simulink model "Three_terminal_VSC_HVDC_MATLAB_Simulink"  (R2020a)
settings: Solver=ode4  StartTime=0.0  StopTime=Tstop  MaxStep=1e-4  RelTol=1e-3
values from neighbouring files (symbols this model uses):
  kw = 5    [Parameterisation_Three_terminal_VSC_HVDC_MATLAB_Simulink.m]
undefined symbols (not defined in the file or in its folder): bridge, phase, pulses, Sim, Three, VSC1, VSC123, VSC2, VSC3
libraries: powerlib x70, powerlib_meascontrol x9, simulink x3
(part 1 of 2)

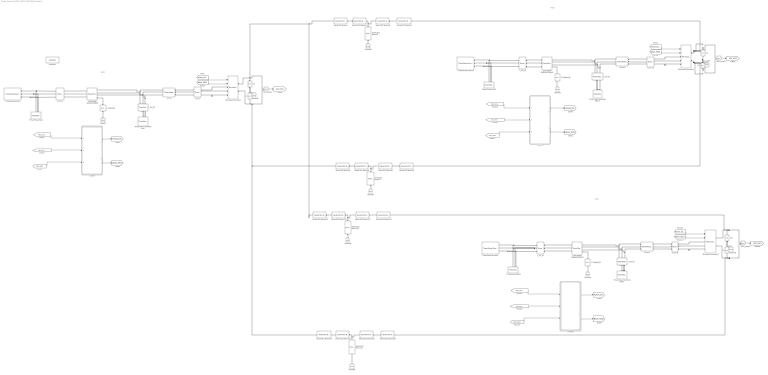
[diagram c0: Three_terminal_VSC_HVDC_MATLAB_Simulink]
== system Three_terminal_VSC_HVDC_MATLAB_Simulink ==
  note: VSC2
  note: VSC3
  note: VSC1
  1.0 [Mohm] : powerlib/Elements/Series RLC Branch  LConnTagsString=__new0  RConnTagsString=__new0  BranchType=R  Resistance=1e6  Inductance=1e-3  SetiL0=off  InitialCurrent=0  Capacitance=1e-6  Setx0=off  InitialVoltage=0  Measurements=None
  1.0 [Mohm]1 : powerlib/Elements/Series RLC Branch  LConnTagsString=__new0  RConnTagsString=__new0  BranchType=R  Resistance=1e6  Inductance=1e-3  SetiL0=off  InitialCurrent=0  Capacitance=1e-6  Setx0=off  InitialVoltage=0  Measurements=None
  1.0 [Mohm]2 : powerlib/Elements/Series RLC Branch  LConnTagsString=__new0  RConnTagsString=__new0  BranchType=R  Resistance=1e6  Inductance=1e-3  SetiL0=off  InitialCurrent=0  Capacitance=1e-6  Setx0=off  InitialVoltage=0  Measurements=None
  1500 [MVA] 420[kV]/230[kV : powerlib/Elements/Three-Phase Transformer (Two Windings)  Winding1Connection=Yg  Winding2Connection=Yn  CoreType=Five-limb core (shell-type)  SetSaturation=off  Hysteresis=off  DataFile='hysteresis'  SetInitialFlux=off  Measurements=None  UNITS=pu  NominalPower=[VSC1.Trf.nominal.MVA,VSC1.Trf.nominal.f]  Winding1=[VSC1.Trf.nominal.HV VSC1.Trf.ur VSC1.Trf.uk]  Winding2=[VSC1.Trf.nominal.LV VSC1.Trf.ur VSC1.Trf.uk]  Rm=VSC1.Trf.MagRm  Lm=VSC1.Trf.MagXm  L0=1.6029  Saturation=[0 0;0.0024 1.2;1 1.52]  InitialFluxes=[0.00087946 -0.00087946 0.00076952]  BreakLoop=off  DiscreteSolver=Trapezoidal iterative  DataType=off  TransfoNumber=1
  1500 [MVA] 420[kV]/230[kV1 : powerlib/Elements/Three-Phase Transformer (Two Windings)  Winding1Connection=Yg  Winding2Connection=Yn  CoreType=Five-limb core (shell-type)  SetSaturation=off  Hysteresis=off  DataFile='hysteresis'  SetInitialFlux=off  Measurements=None  UNITS=pu  NominalPower=[VSC1.Trf.nominal.MVA,VSC2.Trf.nominal.f]  Winding1=[VSC1.Trf.nominal.HV VSC1.Trf.ur VSC1.Trf.uk]  Winding2=[VSC1.Trf.nominal.LV VSC1.Trf.ur VSC1.Trf.uk]  Rm=VSC1.Trf.MagRm  Lm=VSC1.Trf.MagXm  L0=1.6029  Saturation=[0 0;0.0024 1.2;1 1.52]  InitialFluxes=[0.00087946 -0.00087946 0.00076952]  BreakLoop=off  DiscreteSolver=Trapezoidal iterative  DataType=off  TransfoNumber=1
  1500 [MVA] 420[kV]/230[kV2 : powerlib/Elements/Three-Phase Transformer (Two Windings)  Winding1Connection=Yg  Winding2Connection=Yn  CoreType=Five-limb core (shell-type)  SetSaturation=off  Hysteresis=off  DataFile='hysteresis'  SetInitialFlux=off  Measurements=None  UNITS=pu  NominalPower=[VSC1.Trf.nominal.MVA,VSC2.Trf.nominal.f]  Winding1=[VSC3.Trf.nominal.HV VSC1.Trf.ur VSC1.Trf.uk]  Winding2=[VSC1.Trf.nominal.LV VSC1.Trf.ur VSC1.Trf.uk]  Rm=VSC1.Trf.MagRm  Lm=VSC1.Trf.MagXm  L0=1.6029  Saturation=[0 0;0.0024 1.2;1 1.52]  InitialFluxes=[0.00087946 -0.00087946 0.00076952]  BreakLoop=off  DiscreteSolver=Trapezoidal iterative  DataType=off  TransfoNumber=1
  C/1 : powerlib/Elements/Series RLC Branch  LConnTagsString=__new0  RConnTagsString=__new0  BranchType=C  Resistance=0.000001  Inductance=1e-3  SetiL0=off  InitialCurrent=0  Capacitance=VSC1.Capacitor  Setx0=on  InitialVoltage=200e3  Measurements=None
  C/2 : powerlib/Elements/Series RLC Branch  LConnTagsString=__new0  RConnTagsString=__new0  BranchType=RC  Resistance=1e-12  Inductance=1e-3  SetiL0=off  InitialCurrent=0  Capacitance=VSC1.Capacitor  Setx0=on  InitialVoltage=200e3  Measurements=None
  C/3 : powerlib/Elements/Series RLC Branch  LConnTagsString=__new0  RConnTagsString=__new0  BranchType=C  Resistance=0.000001  Inductance=1e-3  SetiL0=off  InitialCurrent=0  Capacitance=VSC1.Capacitor  Setx0=on  InitialVoltage=200e3  Measurements=None
  C/4 : powerlib/Elements/Series RLC Branch  LConnTagsString=__new0  RConnTagsString=__new0  BranchType=RC  Resistance=1e-12  Inductance=1e-3  SetiL0=off  InitialCurrent=0  Capacitance=VSC1.Capacitor  Setx0=on  InitialVoltage=200e3  Measurements=None
  C/5 : powerlib/Elements/Series RLC Branch  LConnTagsString=__new0  RConnTagsString=__new0  BranchType=C  Resistance=0.000001  Inductance=1e-3  SetiL0=off  InitialCurrent=0  Capacitance=VSC1.Capacitor  Setx0=on  InitialVoltage=200e3  Measurements=None
  C/6 : powerlib/Elements/Series RLC Branch  LConnTagsString=__new0  RConnTagsString=__new0  BranchType=RC  Resistance=1e-12  Inductance=1e-3  SetiL0=off  InitialCurrent=0  Capacitance=VSC1.Capacitor  Setx0=on  InitialVoltage=200e3  Measurements=None
  Control : Subsystem
  Control1 : Subsystem
  Control2 : Subsystem
  Ground{,1..9} (10 alike) : powerlib/Elements/Ground  LConnTagsString=a
  I_C/V_C : powerlib/Measurements/Three-Phase V-I Measurement  VoltageMeasurement=no  SetLabelV=off  LabelV=Vabc_converter  Vpu=off  VpuLL=off  CurrentMeasurement=yes  SetLabelI=on  LabelI=Iabc_converter_VSC1  Ipu=off  Pbase=100e6  Vbase=500e3  OutputType=Complex  PhasorSimulation=off  PSBequivalent=0
  I_C/V_C1 : powerlib/Measurements/Three-Phase V-I Measurement  VoltageMeasurement=phase-to-ground  SetLabelV=on  LabelV=Vabc_filter  Vpu=off  VpuLL=off  CurrentMeasurement=yes  SetLabelI=on  LabelI=Iabc_filter  Ipu=off  Pbase=100e6  Vbase=500e3  OutputType=Complex  PhasorSimulation=off  PSBequivalent=0
  I_C/V_C2 : powerlib/Measurements/Three-Phase V-I Measurement  VoltageMeasurement=no  SetLabelV=off  LabelV=Vabc_converter  Vpu=off  VpuLL=off  CurrentMeasurement=yes  SetLabelI=on  LabelI=Iabc_converter_VSC2  Ipu=off  Pbase=100e6  Vbase=500e3  OutputType=Complex  PhasorSimulation=off  PSBequivalent=0
  I_C/V_C3 : powerlib/Measurements/Three-Phase V-I Measurement  VoltageMeasurement=no  SetLabelV=off  LabelV=Vabc_filter  Vpu=off  VpuLL=off  CurrentMeasurement=no  SetLabelI=off  LabelI=Iabc_filter  Ipu=off  Pbase=100e6  Vbase=500e3  OutputType=Complex  PhasorSimulation=off  PSBequivalent=0
  I_C/V_C4 : powerlib/Measurements/Three-Phase V-I Measurement  VoltageMeasurement=no  SetLabelV=off  LabelV=Vabc_converter  Vpu=off  VpuLL=off  CurrentMeasurement=yes  SetLabelI=on  LabelI=Iabc_converter_VSC3  Ipu=off  Pbase=100e6  Vbase=500e3  OutputType=Complex  PhasorSimulation=off  PSBequivalent=0
  I_C/V_C5 : powerlib/Measurements/Three-Phase V-I Measurement  VoltageMeasurement=no  SetLabelV=off  LabelV=Vabc_filter  Vpu=off  VpuLL=off  CurrentMeasurement=no  SetLabelI=off  LabelI=Iabc_filter  Ipu=off  Pbase=100e6  Vbase=500e3  OutputType=Complex  PhasorSimulation=off  PSBequivalent=0
  I_S/V_S : powerlib/Measurements/Three-Phase V-I Measurement  VoltageMeasurement=phase-to-ground  SetLabelV=on  LabelV=Vabc_source_VSC1  Vpu=off  VpuLL=off  CurrentMeasurement=yes  SetLabelI=on  LabelI=Iabc_source_VSC1  Ipu=off  Pbase=100e6  Vbase=500e3  OutputType=Complex  PhasorSimulation=off  PSBequivalent=0
  I_S/V_S1 : powerlib/Measurements/Three-Phase V-I Measurement  VoltageMeasurement=phase-to-ground  SetLabelV=on  LabelV=Vabc_source_VSC2  Vpu=off  VpuLL=off  CurrentMeasurement=yes  SetLabelI=on  LabelI=Iabc_source_VSC2  Ipu=off  Pbase=100e6  Vbase=500e3  OutputType=Complex  PhasorSimulation=off  PSBequivalent=0
  I_S/V_S2 : powerlib/Measurements/Three-Phase V-I Measurement  VoltageMeasurement=phase-to-ground  SetLabelV=on  LabelV=Vabc_source_VSC3  Vpu=off  VpuLL=off  CurrentMeasurement=yes  SetLabelI=on  LabelI=Iabc_source_VSC3  Ipu=off  Pbase=100e6  Vbase=500e3  OutputType=Complex  PhasorSimulation=off  PSBequivalent=0
  LfConv : powerlib/Elements/Three-Phase Series RLC Branch  LConnTagsString=A|B|C  RConnTagsString=A|B|C  BranchType=L  Resistance=1  Inductance=VSC1.SeriesFilter.Lf  Capacitance=1e-6  Measurements=None
  LfConv1 : powerlib/Elements/Three-Phase Series RLC Branch  LConnTagsString=A|B|C  RConnTagsString=A|B|C  BranchType=L  Resistance=1  Inductance=VSC1.SeriesFilter.Lf  Capacitance=1e-6  Measurements=None
  LfConv2 : powerlib/Elements/Three-Phase Series RLC Branch  LConnTagsString=A|B|C  RConnTagsString=A|B|C  BranchType=L  Resistance=1  Inductance=VSC1.SeriesFilter.Lf  Capacitance=1e-6  Measurements=None
  Series RLC Branch{,3,5,8,10,13,15,18} (8 alike) : powerlib/Elements/Series RLC Branch  LConnTagsString=__new0  RConnTagsString=__new0  BranchType=R  Resistance=VSC123.Rline  Inductance=1e-3  SetiL0=off  InitialCurrent=0  Capacitance=1e-6  Setx0=off  InitialVoltage=0  Measurements=None
  Series RLC Branch{1,4,6,9,11,14,16,19} (8 alike) : powerlib/Elements/Series RLC Branch  LConnTagsString=__new0  RConnTagsString=__new0  BranchType=L  Resistance=VSC123.Rline  Inductance=VSC123.Lline  SetiL0=off  InitialCurrent=0  Capacitance=1e-6  Setx0=off  InitialVoltage=0  Measurements=None
  Series RLC Branch{2,7,12,17} (4 alike) : powerlib/Elements/Series RLC Branch  LConnTagsString=__new0  RConnTagsString=__new0  BranchType=C  Resistance=VSC123.Rline  Inductance=VSC123.Lline  SetiL0=off  InitialCurrent=0  Capacitance=VSC123.Cline  Setx0=off  InitialVoltage=0  Measurements=None
  Three-Phase Harmonic Filter : powerlib/Elements/Three-Phase Harmonic Filter  LConnTagsString=A|B|C  FilterType=High-pass  FilterConnection=Y (grounded)  ParNom=[230e3 60]  Qc=75e6  Fr=[450]  Frd=[11*60 13*60]  Q=0.08  Measurements=None
  Three-Phase Harmonic Filter1 : powerlib/Elements/Three-Phase Harmonic Filter  LConnTagsString=A|B|C  FilterType=High-pass  FilterConnection=Y (grounded)  ParNom=[230e3 50]  Qc=75e6  Fr=[450]  Frd=[11*60 13*60]  Q=0.08  Measurements=None
  Three-Phase Harmonic Filter2 : powerlib/Elements/Three-Phase Harmonic Filter  LConnTagsString=A|B|C  FilterType=High-pass  FilterConnection=Y (grounded)  ParNom=[230e3 50]  Qc=75e6  Fr=[450]  Frd=[11*60 13*60]  Q=0.08  Measurements=None
  Three-Phase Fault : powerlib/Elements/Three-Phase Fault  InitialStates=0  FaultA=on  FaultB=on  FaultC=off  GroundFault=on  SwitchTimes="[VSC1.flt.On  VSC1.flt.Off]"  External=off  SwitchStatus=NaN  FaultResistance=VSC1.flt.OnR  GroundResistance=VSC1.flt.GroundR  SnubberResistance=1e6  SnubberCapacitance=inf  Measurements=Fault voltages and currents
  Three-Phase Fault1 : powerlib/Elements/Three-Phase Fault  InitialStates=0  FaultA=on  FaultB=on  FaultC=on  GroundFault=on  SwitchTimes="[VSC2.flt.On  VSC2.flt.Off]"  External=off  SwitchStatus=NaN  FaultResistance=VSC1.flt.OnR  GroundResistance=VSC1.flt.GroundR  SnubberResistance=1e6  SnubberCapacitance=inf  Measurements=Fault voltages and currents
  Three-Phase Fault2 : powerlib/Elements/Three-Phase Fault  InitialStates=0  FaultA=on  FaultB=on  FaultC=on  GroundFault=on  SwitchTimes="[VSC3.flt.On  VSC3.flt.Off]"  External=off  SwitchStatus=NaN  FaultResistance=VSC1.flt.OnR  GroundResistance=VSC1.flt.GroundR  SnubberResistance=1e6  SnubberCapacitance=inf  Measurements=Fault voltages and currents
  Three-Phase Source : powerlib/Electrical Sources/Three-Phase Source  InternalConnection=Yg  VoltagePhases=off  Voltage=VSC1.source.nominal.v  PhaseAngle=VSC1.source.nominal.theta  Voltage_phases=[25e3 25e3 25e3]/sqrt(3)  PhaseAngles_phases=[0 -120 +120]  Frequency=VSC1.source.nominal.f  NonIdealSource=on  SpecifyImpedance=off  Resistance=VSC1.source.nominal.r  Inductance=VSC1.source.nominal.l  ShortCircuitLevel=100e6  BaseVoltage=VSC1.source.basevoltage  XRratio=7  BusType=swing  Pref=10e3  Qref=0  Prefabc=[10e3, 10e3, 10e3]  Qrefabc=[0, 0, 0]  Qmin=-inf  Qmax=inf
  Three-Phase Source1 : powerlib/Electrical Sources/Three-Phase Source  InternalConnection=Yg  VoltagePhases=off  Voltage=VSC1.source.nominal.v  PhaseAngle=VSC1.source.nominal.theta  Voltage_phases=[25e3 25e3 25e3]/sqrt(3)  PhaseAngles_phases=[0 -120 +120]  Frequency=VSC2.source.nominal.f  NonIdealSource=on  SpecifyImpedance=off  Resistance=VSC1.source.nominal.r  Inductance=VSC2.source.nominal.l  ShortCircuitLevel=100e6  BaseVoltage=VSC1.source.basevoltage  XRratio=7  BusType=swing  Pref=10e3  Qref=0  Prefabc=[10e3, 10e3, 10e3]  Qrefabc=[0, 0, 0]  Qmin=-inf  Qmax=inf
  Three-Phase Source2 : powerlib/Electrical Sources/Three-Phase Source  InternalConnection=Yg  VoltagePhases=off  Voltage=VSC3.source.nominal.v  PhaseAngle=VSC1.source.nominal.theta  Voltage_phases=[25e3 25e3 25e3]/sqrt(3)  PhaseAngles_phases=[0 -120 +120]  Frequency=VSC2.source.nominal.f  NonIdealSource=on  SpecifyImpedance=off  Resistance=VSC1.source.nominal.r  Inductance=VSC2.source.nominal.l  ShortCircuitLevel=100e6  BaseVoltage=VSC3.source.nominal.v  XRratio=7  BusType=swing  Pref=10e3  Qref=0  Prefabc=[10e3, 10e3, 10e3]  Qrefabc=[0, 0, 0]  Qmin=-inf  Qmax=inf
  Two-Level Converter : powerlib/Power Electronics/Two-Level Converter  ModelType=Switching devices  Ron=0.005  Rs=1e6  Cs=inf  Vforward=[0,0]  Ron_Diode=1e-3  Rs_Diode=1e6  Cs_Diode=inf  Vf_Diode=1e-3  Rs_CurrentSource=inf
  Two-Level Converter1 : powerlib/Power Electronics/Two-Level Converter  ModelType=Switching devices  Ron=0.005  Rs=1e6  Cs=inf  Vforward=[0,0]  Ron_Diode=1e-3  Rs_Diode=1e6  Cs_Diode=inf  Vf_Diode=1e-3  Rs_CurrentSource=inf
  Two-Level Converter2 : powerlib/Power Electronics/Two-Level Converter  ModelType=Switching devices  Ron=0.005  Rs=1e6  Cs=inf  Vforward=[0,0]  Ron_Diode=1e-3  Rs_Diode=1e6  Cs_Diode=inf  Vf_Diode=1e-3  Rs_CurrentSource=inf
  UDC_meas : powerlib/Measurements/Voltage Measurement  PhasorSimulation=off  OutputType=Complex  PSBequivalent=0
  UDC_meas1 : powerlib/Measurements/Voltage Measurement  PhasorSimulation=off  OutputType=Complex  PSBequivalent=0
  UDC_meas2 : powerlib/Measurements/Voltage Measurement  PhasorSimulation=off  OutputType=Complex  PSBequivalent=0
  powergui : powerlib/powergui  Priority=1  SimulationMode=Discrete  SampleTime=Sim.Ts  frequency=60  Iterations=50  frequencyindice=0  Pbase=100e6  ErrMax=1e-4  UnitsV=kV  UnitsW=MW  buscounter=0  FunctionMessages=off  echomessages=off  EnableUseOfTLC=off  CurrentSourceSwitches=off  DisableSnubberDevices=off  DisableRonSwitches=off  DisableVfSwitches=off  DisplayEquations=off  AutomaticDiscreteSolvers=off  SolverType=Tustin/Backward Euler (TBE)  Interpol=off  ExternalGateDelay=off  methode=off  Ts=100  x0status=blocks  SPID=on  SwTol=0  HookPort=off  NonlinearTolerance=1e-4  nMaxIteration=100  ContinueOnMaxIteration=off  RestoreLinks=warning  ResistiveCurrentMeasurement=off  Frange=[0:2:500]  Ylog=off  Xlog=on  ShowGrid=off  save=off  variable=ZData  structure=0  ZoomFFT=off  StartTime=0.0  cycles=1  DisplayStyle=1  fundamental=60  FreqAxis=off  MaxFrequency=1000  frequencyindicesteady=1  RmsSteady=1  display=off
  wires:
  [Vabc_source_VSC1] -> Control/1(Umeas)
  [Iabc_converter_VSC1] -> Control/2(Imeas)
  Control/1(Pulses) -> [Pulses_VSC1]
  [Pulses_VSC1] -> Two-Level Converter/1
  [Block_VSC1] -> Two-Level Converter/2
  UDC_meas/1 -> [UDC_VSC1]
  [UDC_VSC1] -> Control/3(UDC)
  UDC_meas1/1 -> [UDC_VSC2]
  [Vabc_source_VSC2] -> Control1/1(Umeas)
  [Block_VSC2] -> Two-Level Converter1/2
  [UDC_VSC2] -> Control1/3(UDC)
  [Iabc_converter_VSC2] -> Control1/2(Imeas)
  [Pulses_VSC2] -> Two-Level Converter1/1
  Control1/1(Pulses) -> [Pulses_VSC2]
  [Block_VSC3] -> Two-Level Converter2/2
  UDC_meas2/1 -> [UDC_VSC3]
  [Vabc_source_VSC3] -> Control2/1(Umeas)
  Control2/2("Block ") -> [Block_VSC3]
  [Pulses_VSC3] -> Two-Level Converter2/1
  Control2/1(Pulses) -> [Pulses_VSC3]
  [Iabc_converter_VSC3] -> Control2/2(Imeas)
  [UDC_VSC3] -> Control2/3(UDC)
  Control1/2("Block ") -> [Block_VSC2]
  Control/2("Block ") -> [Block_VSC1]
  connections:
  1.0 [Mohm]/LConn1 -- 1500 [MVA] 420[kV]/230[kV/RConn4
  Ground/LConn1 -- 1.0 [Mohm]/RConn1
  LfConv/RConn1 -- I_C/V_C/LConn1
  LfConv/RConn2 -- I_C/V_C/LConn2
  LfConv/RConn3 -- I_C/V_C/LConn3
  C/2/LConn1 -- UDC_meas/LConn1 -- Series RLC Branch/LConn1 -- Series RLC Branch10/LConn1 -- Two-Level Converter/RConn1
  I_C/V_C1/RConn2 -- LfConv/LConn2 -- 1500 [MVA] 420[kV]/230[kV/RConn2
  I_C/V_C1/RConn3 -- LfConv/LConn3 -- 1500 [MVA] 420[kV]/230[kV/RConn3
  I_C/V_C1/RConn1 -- LfConv/LConn1 -- 1500 [MVA] 420[kV]/230[kV/RConn1
  C/2/RConn1 -- Ground1/LConn1 -- C/1/LConn1
  Three-Phase Source/RConn1 -- Three-Phase Fault/LConn1 -- I_S/V_S/LConn1
  Three-Phase Source/RConn2 -- Three-Phase Fault/LConn2 -- I_S/V_S/LConn2
  Three-Phase Source/RConn3 -- Three-Phase Fault/LConn3 -- I_S/V_S/LConn3
  Series RLC Branch1/LConn1 -- Series RLC Branch/RConn1
  Series RLC Branch2/LConn1 -- Series RLC Branch3/LConn1 -- Series RLC Branch1/RConn1
  Ground6/LConn1 -- Series RLC Branch2/RConn1
  Series RLC Branch4/LConn1 -- Series RLC Branch3/RConn1
  Series RLC Branch7/LConn1 -- Series RLC Branch8/LConn1 -- Series RLC Branch6/RConn1
  Series RLC Branch9/LConn1 -- Series RLC Branch8/RConn1
  Ground7/LConn1 -- Series RLC Branch7/RConn1
  Series RLC Branch6/LConn1 -- Series RLC Branch5/RConn1
  Series RLC Branch12/LConn1 -- Series RLC Branch13/LConn1 -- Series RLC Branch11/RConn1
  Series RLC Branch14/LConn1 -- Series RLC Branch13/RConn1
  Ground8/LConn1 -- Series RLC Branch12/RConn1
  Series RLC Branch11/LConn1 -- Series RLC Branch10/RConn1
  Series RLC Branch17/LConn1 -- Series RLC Branch18/LConn1 -- Series RLC Branch16/RConn1
  Series RLC Branch19/LConn1 -- Series RLC Branch18/RConn1
  Ground9/LConn1 -- Series RLC Branch17/RConn1
  Series RLC Branch16/LConn1 -- Series RLC Branch15/RConn1
  C/3/LConn1 -- C/4/RConn1 -- Ground3/LConn1
  I_C/V_C3/RConn2 -- LfConv1/LConn2 -- 1500 [MVA] 420[kV]/230[kV1/RConn2
  Two-Level Converter1/RConn2 -- UDC_meas1/LConn2 -- Series RLC Branch9/RConn1 -- C/3/RConn1
  I_C/V_C3/RConn1 -- LfConv1/LConn1 -- 1500 [MVA] 420[kV]/230[kV1/RConn1
  Three-Phase Source1/RConn3 -- Three-Phase Fault1/LConn3 -- I_S/V_S1/LConn3
  Two-Level Converter1/RConn1 -- UDC_meas1/LConn1 -- Series RLC Branch4/RConn1 -- C/4/LConn1
  Three-Phase Source1/RConn2 -- Three-Phase Fault1/LConn2 -- I_S/V_S1/LConn2
  Three-Phase Source1/RConn1 -- Three-Phase Fault1/LConn1 -- I_S/V_S1/LConn1
  I_C/V_C3/RConn3 -- 1500 [MVA] 420[kV]/230[kV1/RConn3 -- LfConv1/LConn3
  LfConv1/RConn2 -- I_C/V_C2/LConn2
  LfConv1/RConn3 -- I_C/V_C2/LConn3
  LfConv1/RConn1 -- I_C/V_C2/LConn1
  Ground2/LConn1 -- 1.0 [Mohm]1/RConn1
  1.0 [Mohm]1/LConn1 -- 1500 [MVA] 420[kV]/230[kV1/RConn4
  C/6/RConn1 -- Ground5/LConn1 -- C/5/LConn1
  UDC_meas2/LConn2 -- Series RLC Branch19/RConn1 -- C/5/RConn1 -- Two-Level Converter2/RConn2
  Three-Phase Source2/RConn1 -- Three-Phase Fault2/LConn1 -- I_S/V_S2/LConn1
  UDC_meas2/LConn1 -- C/6/LConn1 -- Series RLC Branch14/RConn1 -- Two-Level Converter2/RConn1
  I_C/V_C5/RConn1 -- LfConv2/LConn1 -- 1500 [MVA] 420[kV]/230[kV2/RConn1
  Three-Phase Source2/RConn3 -- Three-Phase Fault2/LConn3 -- I_S/V_S2/LConn3
  I_C/V_C5/RConn2 -- LfConv2/LConn2 -- 1500 [MVA] 420[kV]/230[kV2/RConn2
  I_C/V_C5/RConn3 -- LfConv2/LConn3 -- 1500 [MVA] 420[kV]/230[kV2/RConn3
  I_S/V_S2/LConn2 -- Three-Phase Source2/RConn2 -- Three-Phase Fault2/LConn2
  LfConv2/RConn2 -- I_C/V_C4/LConn2
  LfConv2/RConn3 -- I_C/V_C4/LConn3
  1.0 [Mohm]2/LConn1 -- 1500 [MVA] 420[kV]/230[kV2/RConn4
  Ground4/LConn1 -- 1.0 [Mohm]2/RConn1
  LfConv2/RConn1 -- I_C/V_C4/LConn1
  1500 [MVA] 420[kV]/230[kV/LConn1 -- I_S/V_S/RConn1
  1500 [MVA] 420[kV]/230[kV/LConn2 -- I_S/V_S/RConn2
  1500 [MVA] 420[kV]/230[kV/LConn3 -- I_S/V_S/RConn3
  1500 [MVA] 420[kV]/230[kV2/LConn1 -- I_S/V_S2/RConn1
  1500 [MVA] 420[kV]/230[kV2/LConn2 -- I_S/V_S2/RConn2
  1500 [MVA] 420[kV]/230[kV2/LConn3 -- I_S/V_S2/RConn3
  1500 [MVA] 420[kV]/230[kV1/LConn1 -- I_S/V_S1/RConn1
  I_S/V_S1/RConn2 -- 1500 [MVA] 420[kV]/230[kV1/LConn2
  I_S/V_S1/RConn3 -- 1500 [MVA] 420[kV]/230[kV1/LConn3
  Three-Phase Harmonic Filter/LConn1 -- I_C/V_C1/LConn1
  Three-Phase Harmonic Filter/LConn2 -- I_C/V_C1/LConn2
  Three-Phase Harmonic Filter/LConn3 -- I_C/V_C1/LConn3
  Three-Phase Harmonic Filter1/LConn1 -- I_C/V_C3/LConn1
  I_C/V_C3/LConn2 -- Three-Phase Harmonic Filter1/LConn2
  Three-Phase Harmonic Filter1/LConn3 -- I_C/V_C3/LConn3
  Three-Phase Harmonic Filter2/LConn1 -- I_C/V_C5/LConn1
  Three-Phase Harmonic Filter2/LConn2 -- I_C/V_C5/LConn2
  Three-Phase Harmonic Filter2/LConn3 -- I_C/V_C5/LConn3
  UDC_meas/LConn2 -- Series RLC Branch15/LConn1 -- Series RLC Branch5/LConn1 -- C/1/RConn1 -- Two-Level Converter/RConn2
  I_C/V_C/RConn1 -- Two-Level Converter/LConn1
  I_C/V_C/RConn2 -- Two-Level Converter/LConn2
  I_C/V_C/RConn3 -- Two-Level Converter/LConn3
  I_C/V_C2/RConn1 -- Two-Level Converter1/LConn1
  I_C/V_C2/RConn2 -- Two-Level Converter1/LConn2
  I_C/V_C2/RConn3 -- Two-Level Converter1/LConn3
  I_C/V_C4/RConn1 -- Two-Level Converter2/LConn1
  I_C/V_C4/RConn2 -- Two-Level Converter2/LConn2
  I_C/V_C4/RConn3 -- Two-Level Converter2/LConn3

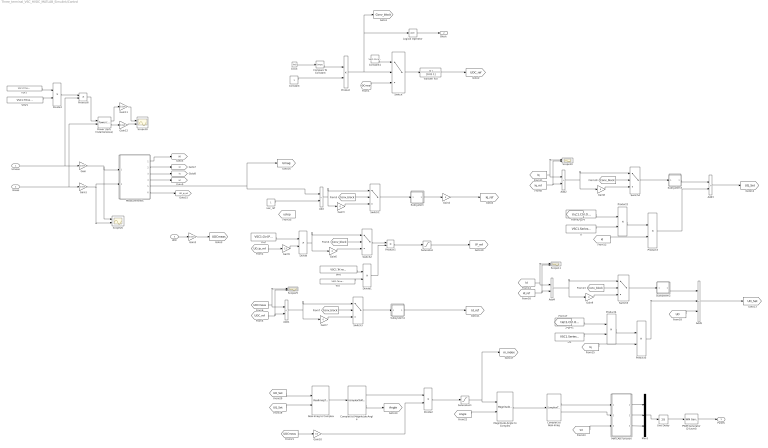
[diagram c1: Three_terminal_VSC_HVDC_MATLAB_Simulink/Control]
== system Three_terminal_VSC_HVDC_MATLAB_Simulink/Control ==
  Umeas : Inport
  Imeas : Inport  Port=2
  UDC : Inport  Port=3
  2*pi*f : Constant  Value=VSC1.Ctrl.Omeganom
  2*pi*f1 : Constant  Value=VSC1.Ctrl.Omeganom
  Add{,1..4} (5 alike) : Sum  Inputs=-+
  Add5 : Sum  Inputs=--+
  Clock : Clock
  Compare To Constant : simulink/Logic and Bit Operations/Compare To Constant  relop=>  const=0.05  OutDataTypeStr=boolean
  Complex to Magnitude-Angle : ComplexToMagnitudeAngle
  Complex to Real-Imag : ComplexToRealImag
  Constant : Constant
  Constant1 : Constant  Value=VSC1.Ctrl.UDCRef_Const
  Divide{,1..3} (4 alike) : Product  Inputs=*/
  Gain : Gain  Gain=1/1e3
  Gain1 : Gain  Gain=1/1e3
  Gain10 : Gain  Gain=0.5
  Gain11 : Gain  Gain=1/1e6
  Gain12 : Gain  Gain=1/1e6
  Gain2 : Gain  Gain=1/1e3
  Gain{3,6..9} (5 alike) : Gain  Gain=0
  Gain4 : Gain
  Gain5 : Gain  Gain=1.5
  Lf : Constant  Value=VSC1.SeriesFilter.Lf
  Lf1 : Constant  Value=VSC1.SeriesFilter.Lf
  Logical Operator : Logic  Operator=NOT  AllPortsSameDT=off  OutDataTypeStr=boolean
  MATLAB Function : MATLAB Function  TreatAsAtomicUnit=on
  Magnitude-Angle to Complex : MagnitudeAngleToComplex
  Measurements : Subsystem
  Mux1 : Mux  Inputs=3
  PWM Generator (2-Level) : powerlib_meascontrol/Pulse & Signal Generators/PWM Generator (2-Level)  ModulatorType=Three-phase bridge (6 pulses)  ModulatorMode=Unsynchronized  Fc=VSC1.Ctrl.fs  Pc=90  nF=33  MinMax="[ -1  1]"  SamplingTechnique=Natural  ModulatingSignals=off  m=0.8  Freq=60  Phase=0  Ts=Sim.Ts  ShowCarrierOutport=off
  "Power (3ph, Instantaneous)" : powerlib_meascontrol/Measurements/Power (3ph, Instantaneous)
  Pref : Constant  Value=VSC1.Ctrl.Pref
  Product{,1..6} (7 alike) : Product
  Real-Imag to Complex : RealImagToComplex
  Saturation : Saturate  UpperLimit=VSC1.Ctrl.Idmax  LowerLimit=VSC1.Ctrl.Idmin
  Saturation1 : Saturate  UpperLimit=1.1  LowerLimit=0
  Scope{10..11,18,25..26} (5 alike) : Scope  NumInputPorts=2
  Subsystem : Subsystem
  Subsystem1 : Subsystem
  Subsystem2 : Subsystem
  Subsystem3 : Subsystem
  Switch{,1..5} (6 alike) : Switch  Threshold=1
  Transfer Fcn : TransferFcn  Denominator=[0.01 1]
  Unit Delay : UnitDelay  SampleTime=Sim.Ts  HasFrameUpgradeWarning=on
  VHV : Constant  Value=VSC1.Trf.nominal.HV
  VHV1 : Constant  Value=VSC1.Trf.nominal.HV
  VLV : Constant  Value=VSC1.Trf.nominal.LV
  VLV1 : Constant  Value=VSC1.Trf.nominal.LV
  uac_ref : Constant
  Pulses : Outport
  "Block " : Outport  Port=2
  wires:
  Umeas/1 -> Product6/2, Gain/1
  Gain/1 -> Scope26/1, Measurements/1(Umeas)
  Gain1/1 -> Scope26/2, Measurements/2(Imeas)
  UDC/1 -> Gain2/1
  Gain2/1 -> [UDCmeas]
  Add/1 -> Switch1/1, Gain3/1
  Gain3/1 -> Switch1/3
  [Conv_block] -> Switch1/2
  Switch1/1 -> Subsystem/1(Input)
  Subsystem/1(Output) -> Gain4/1
  Gain4/1 -> [Iq_ref]
  Pref/1 -> Divide/1
  Measurements/1(UD) -> [UD]
  Measurements/2(Id) -> [Id]
  Measurements/3(Iq) -> [Iq]
  Measurements/4(Phi) -> [wt]
  [UD_ip_ref] -> Gain5/1
  Gain5/1 -> Divide/2
  [Conv_block] -> Switch2/2
  Gain6/1 -> Switch2/3
  Divide/1 -> Gain6/1, Switch2/1
  VLV/1 -> Divide1/2
  VHV/1 -> Divide1/1
  Switch2/1 -> Product1/1
  Divide1/1 -> Product1/2
  Product1/1 -> Saturation/1
  Saturation/1 -> [IP_ref]
  [UDC_ref] -> Scope25/2, Add1/2
  Gain7/1 -> Switch3/3
  Add1/1 -> Gain7/1, Switch3/1
  [Conv_block] -> Switch3/2
  Switch3/1 -> Subsystem1/1(Input)
  Subsystem1/1(Output) -> [Id_ref]
  [Conv_block] -> Switch4/2
  [Iq_ref] -> Scope10/2, Add2/2
  Gain8/1 -> Switch4/3
  Add2/1 -> Gain8/1, Switch4/1
  Subsystem3/1(Output) -> Add3/1
  2*pi*f/1 -> Product2/1
  Lf/1 -> Product2/2
  Product2/1 -> Product3/1
  [Iq] -> Scope10/1, Add2/1
  [Id] -> Product3/2
  Product3/1 -> Add3/2
  Add3/1 -> [UQ_Set]
  Lf1/1 -> Product4/2
  [Id] -> Scope11/1, Add4/1
  2*pi*f1/1 -> Product4/1
  Switch5/1 -> Subsystem2/1(Input)
  Product4/1 -> Product5/1
  [Id_ref] -> Scope11/2, Add4/2
  [Conv_block] -> Switch5/2
  [Iq] -> Product5/2
  Product5/1 -> Add5/2
  Gain9/1 -> Switch5/3
  Add5/1 -> [UD_Set]
  Add4/1 -> Gain9/1, Switch5/1
  Subsystem2/1(Output) -> Add5/1
  [UQ_Set] -> Real-Imag to Complex/2
  [UD_Set] -> Real-Imag to Complex/1
  Real-Imag to Complex/1 -> Complex to Magnitude-Angle/1
  Complex to Magnitude-Angle/1 -> Divide2/1
  Gain10/1 -> Divide2/2
  Divide2/1 -> Saturation1/1
  Complex to Magnitude-Angle/2 -> [Angle]
  [Angle] -> Magnitude-Angle to Complex/2
  Magnitude-Angle to Complex/1 -> Complex to Real-Imag/1
  Complex to Real-Imag/1 -> MATLAB Function/1(Pmd)
  Complex to Real-Imag/2 -> MATLAB Function/2(Pmq)
  Switch4/1 -> Subsystem3/1(Input)
  "Power (3ph, Instantaneous)"/1 -> Gain11/1
  "Power (3ph, Instantaneous)"/2 -> Gain12/1
  Gain11/1 -> Scope18/1
  Gain12/1 -> Scope18/2
  [UDCmeas] -> Scope25/1, Add1/1
  [UD] -> Add5/3
  Measurements/6(UD_ip_ref) -> [UD_ip_ref]
  Divide3/1 -> Product6/1
  Product6/1 -> "Power (3ph, Instantaneous)"/1
  Imeas/1 -> "Power (3ph, Instantaneous)"/2, Gain1/1
  VLV1/1 -> Divide3/1
  VHV1/1 -> Divide3/2
  Measurements/5(Umag) -> Add/1, [Umag]
  Saturation1/1 -> [m_index], Magnitude-Angle to Complex/1
  [wt] -> MATLAB Function/3(theta)
  MATLAB Function/1(xA) -> Mux1/1
  MATLAB Function/2(xB) -> Mux1/2
  MATLAB Function/3(xC) -> Mux1/3
  Mux1/1 -> Unit Delay/1
  Unit Delay/1 -> PWM Generator (2-Level)/1
  uac_ref/1 -> Add/2
  PWM Generator (2-Level)/1 -> Pulses/1
  [UDCmeas] -> Gain10/1
  Transfer Fcn/1 -> [UDC_ref]
  Logical Operator/1 -> "Block "/1
  Constant1/1 -> Switch/1
  Product/1 -> Logical Operator/1, [Conv_block], Switch/2
  Compare To Constant/1 -> Product/1
  Clock/1 -> Compare To Constant/1
  Constant/1 -> Product/2
  [UDCmeas] -> Switch/3
  Switch/1 -> Transfer Fcn/1

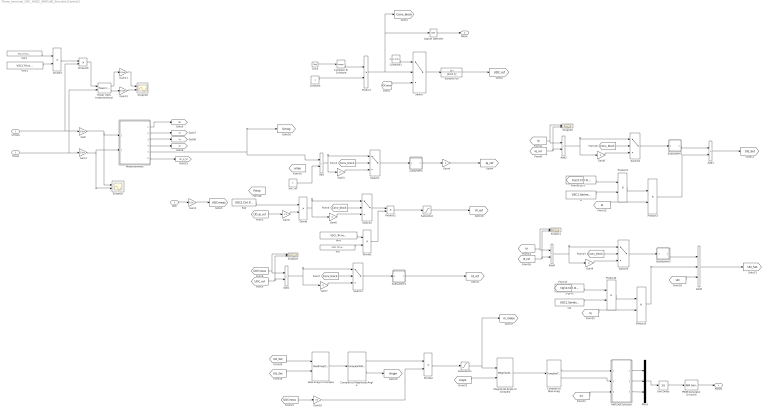
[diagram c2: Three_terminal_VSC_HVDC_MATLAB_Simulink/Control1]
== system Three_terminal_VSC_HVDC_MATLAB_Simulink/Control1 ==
  Umeas : Inport
  Imeas : Inport  Port=2
  UDC : Inport  Port=3
  2*pi*f : Constant  Value=VSC2.Ctrl.Omeganom
  2*pi*f1 : Constant  Value=VSC2.Ctrl.Omeganom
  Add{,1..4} (5 alike) : Sum  Inputs=-+
  Add5 : Sum  Inputs=--+
  Clock : Clock
  Compare To Constant : simulink/Logic and Bit Operations/Compare To Constant  relop=>  const=0.05  OutDataTypeStr=boolean
  Complex to Magnitude-Angle : ComplexToMagnitudeAngle
  Complex to Real-Imag : ComplexToRealImag
  Constant : Constant
  Constant1 : Constant  Value=VSC1.Ctrl.UDCRef_Const
  Divide{,1..3} (4 alike) : Product  Inputs=*/
  Gain : Gain  Gain=1/1e3
  Gain1 : Gain  Gain=1/1e3
  Gain10 : Gain  Gain=0.5
  Gain11 : Gain  Gain=1/1e6
  Gain12 : Gain  Gain=1/1e6
  Gain2 : Gain  Gain=1/1e3
  Gain{3,6..9} (5 alike) : Gain  Gain=0
  Gain4 : Gain
  Gain5 : Gain  Gain=1.5
  Lf : Constant  Value=VSC1.SeriesFilter.Lf
  Lf1 : Constant  Value=VSC1.SeriesFilter.Lf
  Logical Operator : Logic  Operator=NOT  AllPortsSameDT=off  OutDataTypeStr=boolean
  MATLAB Function : MATLAB Function  TreatAsAtomicUnit=on
  Magnitude-Angle to Complex : MagnitudeAngleToComplex
  Measurements : Subsystem
  Mux1 : Mux  Inputs=3
  PWM Generator (2-Level) : powerlib_meascontrol/Pulse & Signal Generators/PWM Generator (2-Level)  ModulatorType=Three-phase bridge (6 pulses)  ModulatorMode=Unsynchronized  Fc=VSC1.Ctrl.fs  Pc=90  nF=33  MinMax="[ -1  1]"  SamplingTechnique=Natural  ModulatingSignals=off  m=0.8  Freq=60  Phase=0  Ts=Sim.Ts  ShowCarrierOutport=off
  "Power (3ph, Instantaneous)" : powerlib_meascontrol/Measurements/Power (3ph, Instantaneous)
  Pref : Constant  Value=VSC2.Ctrl.Pref
  Product{,1..6} (7 alike) : Product
  Real-Imag to Complex : RealImagToComplex
  Saturation : Saturate  UpperLimit=VSC1.Ctrl.Idmax  LowerLimit=VSC1.Ctrl.Idmin
  Saturation1 : Saturate  UpperLimit=1.1  LowerLimit=0
  Scope{10..11,18,25..26} (5 alike) : Scope  NumInputPorts=2
  Subsystem : Subsystem
  Subsystem1 : Subsystem
  Subsystem2 : Subsystem
  Subsystem3 : Subsystem
  Switch{,1..5} (6 alike) : Switch  Threshold=1
  Transfer Fcn : TransferFcn  Denominator=[0.01 1]
  Unit Delay : UnitDelay  SampleTime=Sim.Ts  HasFrameUpgradeWarning=on
  VHV : Constant  Value=VSC1.Trf.nominal.HV
  VHV1 : Constant  Value=VSC1.Trf.nominal.HV
  VLV : Constant  Value=VSC1.Trf.nominal.LV
  VLV1 : Constant  Value=VSC1.Trf.nominal.LV
  uac_ref : Constant
  Pulses : Outport
  "Block " : Outport  Port=2
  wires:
  Umeas/1 -> Product6/2, Gain/1
  Gain/1 -> Scope26/1, Measurements/1(Umeas)
  Gain1/1 -> Scope26/2, Measurements/2(Imeas)
  UDC/1 -> Gain2/1
  Gain2/1 -> [UDCmeas]
  Add/1 -> Switch1/1, Gain3/1
  Gain3/1 -> Switch1/3
  [Conv_block] -> Switch1/2
  Switch1/1 -> Subsystem/1(Input)
  Subsystem/1(Output) -> Gain4/1
  Gain4/1 -> [Iq_ref]
  Measurements/1(UD) -> [UD]
  Measurements/2(Id) -> [Id]
  Measurements/3(Iq) -> [Iq]
  Measurements/4(Phi) -> [wt]
  [UD_ip_ref] -> Gain5/1
  Gain5/1 -> Divide/2
  [Conv_block] -> Switch2/2
  Gain6/1 -> Switch2/3
  Divide/1 -> Gain6/1, Switch2/1
  VLV/1 -> Divide1/2
  VHV/1 -> Divide1/1
  Switch2/1 -> Product1/1
  Divide1/1 -> Product1/2
  Product1/1 -> Saturation/1
  Saturation/1 -> [IP_ref]
  [UDC_ref] -> Scope25/2, Add1/2
  Gain7/1 -> Switch3/3
  Add1/1 -> Gain7/1, Switch3/1
  [Conv_block] -> Switch3/2
  Switch3/1 -> Subsystem1/1(Input)
  Subsystem1/1(Output) -> [Id_ref]
  [Conv_block] -> Switch4/2
  [Iq_ref] -> Scope10/2, Add2/2
  Gain8/1 -> Switch4/3
  Add2/1 -> Gain8/1, Switch4/1
  Subsystem2/1(Output) -> Add3/1
  2*pi*f/1 -> Product2/1
  Lf/1 -> Product2/2
  Product2/1 -> Product3/1
  [Iq] -> Scope10/1, Add2/1
  [Id] -> Product3/2
  Product3/1 -> Add3/2
  Add3/1 -> [UQ_Set]
  Lf1/1 -> Product4/2
  [Id] -> Scope11/1, Add4/1
  2*pi*f1/1 -> Product4/1
  Switch5/1 -> Subsystem3/1(Input)
  Product4/1 -> Product5/1
  [IP_ref] -> Scope11/2, Add4/2
  [Conv_block] -> Switch5/2
  [Iq] -> Product5/2
  Product5/1 -> Add5/2
  Gain9/1 -> Switch5/3
  Add5/1 -> [UD_Set]
  Add4/1 -> Gain9/1, Switch5/1
  Subsystem3/1(Output) -> Add5/1
  [UQ_Set] -> Real-Imag to Complex/2
  [UD_Set] -> Real-Imag to Complex/1
  Real-Imag to Complex/1 -> Complex to Magnitude-Angle/1
  [UDCmeas] -> Gain10/1
  Complex to Magnitude-Angle/1 -> Divide2/1
  Gain10/1 -> Divide2/2
  Divide2/1 -> Saturation1/1
  Complex to Magnitude-Angle/2 -> [Angle]
  [Angle] -> Magnitude-Angle to Complex/2
  Magnitude-Angle to Complex/1 -> Complex to Real-Imag/1
  Complex to Real-Imag/1 -> MATLAB Function/1(Pmd)
  Complex to Real-Imag/2 -> MATLAB Function/2(Pmq)
  Switch4/1 -> Subsystem2/1(Input)
  "Power (3ph, Instantaneous)"/1 -> Gain11/1
  "Power (3ph, Instantaneous)"/2 -> Gain12/1
  Unit Delay/1 -> PWM Generator (2-Level)/1
  Gain11/1 -> Scope18/1
  Gain12/1 -> Scope18/2
  [UDCmeas] -> Scope25/1, Add1/1
  [UD] -> Add5/3
  Measurements/6(UD_ip_ref) -> [UD_ip_ref]
  Divide3/1 -> Product6/1
  Product6/1 -> "Power (3ph, Instantaneous)"/1
  Imeas/1 -> "Power (3ph, Instantaneous)"/2, Gain1/1
  VLV1/1 -> Divide3/1
  VHV1/1 -> Divide3/2
  Measurements/5(Umag) -> Add/1, [Umag]
  Saturation1/1 -> [m_index], Magnitude-Angle to Complex/1
  [wt] -> MATLAB Function/3(theta)
  MATLAB Function/1(xA) -> Mux1/1
  MATLAB Function/2(xB) -> Mux1/2
  MATLAB Function/3(xC) -> Mux1/3
  Mux1/1 -> Unit Delay/1
  uac_ref/1 -> Add/2
  Pref/1 -> Divide/1
  PWM Generator (2-Level)/1 -> Pulses/1
  Compare To Constant/1 -> Product/1
  Constant1/1 -> Switch/1
  Switch/1 -> Transfer Fcn/1
  [UDCmeas] -> Switch/3
  Product/1 -> Logical Operator/1, [Conv_block], Switch/2
  Constant/1 -> Product/2
  Clock/1 -> Compare To Constant/1
  Logical Operator/1 -> "Block "/1
  Transfer Fcn/1 -> [UDC_ref]

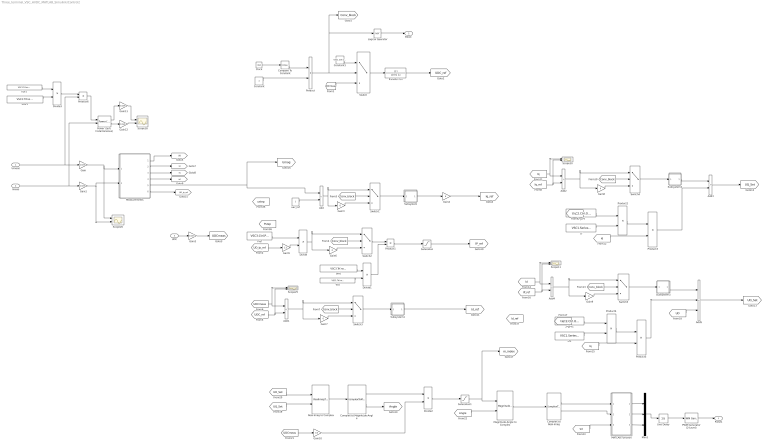
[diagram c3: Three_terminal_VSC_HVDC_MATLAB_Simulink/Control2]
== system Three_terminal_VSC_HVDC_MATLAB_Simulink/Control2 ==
  Umeas : Inport
  Imeas : Inport  Port=2
  UDC : Inport  Port=3
  2*pi*f : Constant  Value=VSC2.Ctrl.Omeganom
  2*pi*f1 : Constant  Value=VSC2.Ctrl.Omeganom
  Add{,1..4} (5 alike) : Sum  Inputs=-+
  Add5 : Sum  Inputs=--+
  Clock : Clock
  Compare To Constant : simulink/Logic and Bit Operations/Compare To Constant  relop=>  const=0.05  OutDataTypeStr=boolean
  Complex to Magnitude-Angle : ComplexToMagnitudeAngle
  Complex to Real-Imag : ComplexToRealImag
  Constant : Constant
  Constant1 : Constant  Value=VSC1.Ctrl.UDCRef_Const
  Divide{,1..3} (4 alike) : Product  Inputs=*/
  Gain : Gain  Gain=1/1e3
  Gain1 : Gain  Gain=1/1e3
  Gain10 : Gain  Gain=0.5
  Gain11 : Gain  Gain=1/1e6
  Gain12 : Gain  Gain=1/1e6
  Gain2 : Gain  Gain=1/1e3
  Gain{3,6..9} (5 alike) : Gain  Gain=0
  Gain4 : Gain
  Gain5 : Gain  Gain=1.5
  Lf : Constant  Value=VSC1.SeriesFilter.Lf
  Lf1 : Constant  Value=VSC1.SeriesFilter.Lf
  Logical Operator : Logic  Operator=NOT  AllPortsSameDT=off  OutDataTypeStr=boolean
  MATLAB Function : MATLAB Function  TreatAsAtomicUnit=on
  Magnitude-Angle to Complex : MagnitudeAngleToComplex
  Measurements : Subsystem
  Mux1 : Mux  Inputs=3
  PWM Generator (2-Level) : powerlib_meascontrol/Pulse & Signal Generators/PWM Generator (2-Level)  ModulatorType=Three-phase bridge (6 pulses)  ModulatorMode=Unsynchronized  Fc=VSC1.Ctrl.fs  Pc=90  nF=33  MinMax="[ -1  1]"  SamplingTechnique=Natural  ModulatingSignals=off  m=0.8  Freq=60  Phase=0  Ts=Sim.Ts  ShowCarrierOutport=off
  "Power (3ph, Instantaneous)" : powerlib_meascontrol/Measurements/Power (3ph, Instantaneous)
  Pref : Constant  Value=VSC3.Ctrl.Pref
  Product{,1..6} (7 alike) : Product
  Real-Imag to Complex : RealImagToComplex
  Saturation : Saturate  UpperLimit=VSC1.Ctrl.Idmax  LowerLimit=VSC1.Ctrl.Idmin
  Saturation1 : Saturate  UpperLimit=1.1  LowerLimit=0
  Scope{10..11,18,25..26} (5 alike) : Scope  NumInputPorts=2
  Subsystem : Subsystem
  Subsystem1 : Subsystem
  Subsystem2 : Subsystem
  Subsystem3 : Subsystem
  Switch{,1..5} (6 alike) : Switch  Threshold=1
  Transfer Fcn : TransferFcn  Denominator=[0.01 1]
  Unit Delay : UnitDelay  SampleTime=Sim.Ts  HasFrameUpgradeWarning=on
  VHV : Constant  Value=VSC3.Trf.nominal.HV
  VHV1 : Constant  Value=VSC3.Trf.nominal.HV
  VLV : Constant  Value=VSC1.Trf.nominal.LV
  VLV1 : Constant  Value=VSC1.Trf.nominal.LV
  uac_ref : Constant
  Pulses : Outport
  "Block " : Outport  Port=2
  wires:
  Clock/1 -> Compare To Constant/1
  Compare To Constant/1 -> Product/1
  Constant/1 -> Product/2
  Product/1 -> Logical Operator/1, [Conv_block], Switch/2
  [UDCmeas] -> Switch/3
  Constant1/1 -> Switch/1
  Switch/1 -> Transfer Fcn/1
  Logical Operator/1 -> "Block "/1
  Umeas/1 -> Product6/2, Gain/1
  Gain/1 -> Scope26/1, Measurements/1(Umeas)
  Gain1/1 -> Scope26/2, Measurements/2(Imeas)
  UDC/1 -> Gain2/1
  Gain2/1 -> [UDCmeas]
  Transfer Fcn/1 -> [UDC_ref]
  Add/1 -> Switch1/1, Gain3/1
  Gain3/1 -> Switch1/3
  [Conv_block] -> Switch1/2
  Switch1/1 -> Subsystem/1(Input)
  Subsystem/1(Output) -> Gain4/1
  Gain4/1 -> [Iq_ref]
  Measurements/1(UD) -> [UD]
  Measurements/2(Id) -> [Id]
  Measurements/3(Iq) -> [Iq]
  Measurements/4(Phi) -> [wt]
  [UD_ip_ref] -> Gain5/1
  Gain5/1 -> Divide/2
  [Conv_block] -> Switch2/2
  Gain6/1 -> Switch2/3
  Divide/1 -> Gain6/1, Switch2/1
  VLV/1 -> Divide1/2
  VHV/1 -> Divide1/1
  Switch2/1 -> Product1/1
  Divide1/1 -> Product1/2
  Product1/1 -> Saturation/1
  Saturation/1 -> [IP_ref]
  [UDC_ref] -> Scope25/2, Add1/2
  Gain7/1 -> Switch3/3
  Add1/1 -> Gain7/1, Switch3/1
  [Conv_block] -> Switch3/2
  Switch3/1 -> Subsystem1/1(Input)
  Subsystem1/1(Output) -> [Id_ref]
  [Conv_block] -> Switch4/2
  [Iq_ref] -> Scope10/2, Add2/2
  Gain8/1 -> Switch4/3
  Add2/1 -> Gain8/1, Switch4/1
  Subsystem2/1(Output) -> Add3/1
  2*pi*f/1 -> Product2/1
  Lf/1 -> Product2/2
  Product2/1 -> Product3/1
  [Iq] -> Scope10/1, Add2/1
  [Id] -> Product3/2
  Product3/1 -> Add3/2
  Add3/1 -> [UQ_Set]
  Lf1/1 -> Product4/2
  [Id] -> Scope11/1, Add4/1
  2*pi*f1/1 -> Product4/1
  Switch5/1 -> Subsystem3/1(Input)
  Product4/1 -> Product5/1
  [Conv_block] -> Switch5/2
  [Iq] -> Product5/2
  Product5/1 -> Add5/2
  Gain9/1 -> Switch5/3
  Add5/1 -> [UD_Set]
  Add4/1 -> Gain9/1, Switch5/1
  Subsystem3/1(Output) -> Add5/1
  [UQ_Set] -> Real-Imag to Complex/2
  [UD_Set] -> Real-Imag to Complex/1
  Real-Imag to Complex/1 -> Complex to Magnitude-Angle/1
  [UDCmeas] -> Gain10/1
  Complex to Magnitude-Angle/1 -> Divide2/1
  Gain10/1 -> Divide2/2
  Divide2/1 -> Saturation1/1
  Complex to Magnitude-Angle/2 -> [Angle]
  [Angle] -> Magnitude-Angle to Complex/2
  Magnitude-Angle to Complex/1 -> Complex to Real-Imag/1
  Complex to Real-Imag/1 -> MATLAB Function/1(Pmd)
  Complex to Real-Imag/2 -> MATLAB Function/2(Pmq)
  Switch4/1 -> Subsystem2/1(Input)
  "Power (3ph, Instantaneous)"/1 -> Gain11/1
  "Power (3ph, Instantaneous)"/2 -> Gain12/1
  Unit Delay/1 -> PWM Generator (2-Level)/1
  Gain11/1 -> Scope18/1
  Gain12/1 -> Scope18/2
  [UDCmeas] -> Scope25/1, Add1/1
  [UD] -> Add5/3
  Measurements/6(UD_ip_ref) -> [UD_ip_ref]
  Divide3/1 -> Product6/1
  Product6/1 -> "Power (3ph, Instantaneous)"/1
  Imeas/1 -> "Power (3ph, Instantaneous)"/2, Gain1/1
  VLV1/1 -> Divide3/1
  VHV1/1 -> Divide3/2
  Measurements/5(Umag) -> Add/1, [Umag]
  Saturation1/1 -> [m_index], Magnitude-Angle to Complex/1
  [wt] -> MATLAB Function/3(theta)
  MATLAB Function/1(xA) -> Mux1/1
  MATLAB Function/2(xB) -> Mux1/2
  MATLAB Function/3(xC) -> Mux1/3
  Mux1/1 -> Unit Delay/1
  uac_ref/1 -> Add/2
  Pref/1 -> Divide/1
  [IP_ref] -> Scope11/2, Add4/2
  PWM Generator (2-Level)/1 -> Pulses/1

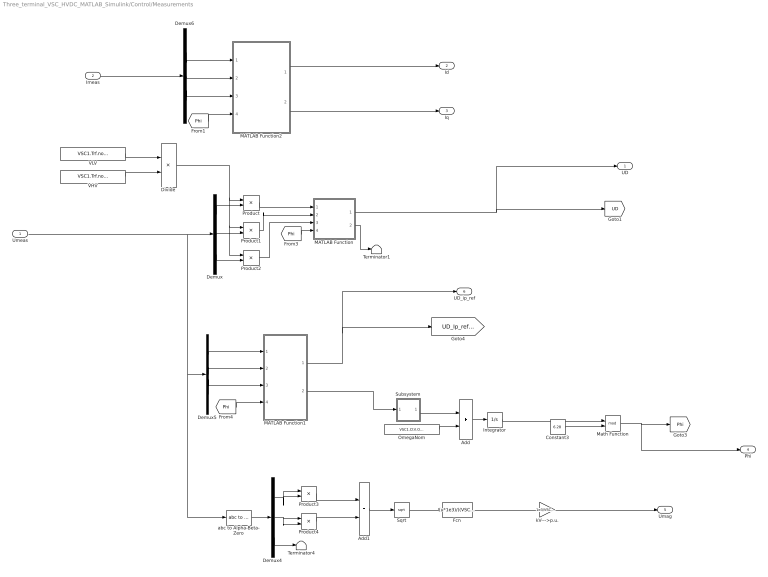
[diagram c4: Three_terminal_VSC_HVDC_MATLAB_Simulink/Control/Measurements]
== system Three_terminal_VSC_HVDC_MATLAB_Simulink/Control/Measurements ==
  Umeas : Inport
  Imeas : Inport  Port=2
  Add : Sum
  Add1 : Sum
  Constant3 : Constant  Value=6.28
  Demux{,4..6} (4 alike) : Demux  Outputs=3
  Divide : Product  Inputs=*/
  Fcn : Fcn  Expr=(u*1e3)/((VSC1.Trf.nominal.HV *sqrt(2))/(sqrt(3)*VSC1.Trf.nominal.HV ))/1000
  Integrator : Integrator
  MATLAB Function : MATLAB Function  TreatAsAtomicUnit=on
  MATLAB Function1 : MATLAB Function  TreatAsAtomicUnit=on
  MATLAB Function2 : MATLAB Function  TreatAsAtomicUnit=on
  Math Function : Math  Operator=mod
  OmegaNom : Constant  Value=VSC1.Ctrl.Omeganom
  Product{,1..4} (5 alike) : Product
  Sqrt : Sqrt
  Subsystem : Subsystem
  Terminator1 : Terminator
  Terminator4 : Terminator
  VHV : Constant  Value=VSC1.Trf.nominal.HV
  VLV : Constant  Value=VSC1.Trf.nominal.LV
  abc to Alpha-Beta-Zero : powerlib_meascontrol/Transformations/abc to Alpha-Beta-Zero
  kV--->p.u. : Gain  Gain=1e3/VSC1.Trf.nominal.HV
  UD : Outport
  Id : Outport  Port=2
  Iq : Outport  Port=3
  Phi : Outport  Port=4
  Umag : Outport  Port=5
  UD_ip_ref : Outport  Port=6
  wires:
  MATLAB Function1/2(xQ) -> Subsystem/1(Input)
  MATLAB Function2/2(xQ) -> Iq/1
  Demux/2 -> Product1/2
  Subsystem/1(Output) -> Add/1
  Math Function/1 -> Phi/1, [Phi]
  Product2/1 -> MATLAB Function/3(xC)
  Divide/1 -> Product/1, Product1/1, Product2/1
  Product/1 -> MATLAB Function/1(xA)
  VLV/1 -> Divide/1
  OmegaNom/1 -> Add/2
  Product1/1 -> MATLAB Function/2(xB)
  Add/1 -> Integrator/1
  VHV/1 -> Divide/2
  Demux/1 -> Product/2
  Demux/3 -> Product2/2
  MATLAB Function2/1(xD) -> Id/1
  abc to Alpha-Beta-Zero/1 -> Demux4/1
  Demux4/1 -> Product3/2, Product3/1
  Demux4/2 -> Product4/2, Product4/1
  Demux4/3 -> Terminator4/1
  Product3/1 -> Add1/1
  Product4/1 -> Add1/2
  Add1/1 -> Sqrt/1
  Sqrt/1 -> Fcn/1
  Fcn/1 -> kV--->p.u./1
  kV--->p.u./1 -> Umag/1
  Umeas/1 -> Demux/1, abc to Alpha-Beta-Zero/1, Demux5/1
  MATLAB Function1/1(xD) -> [UD_Ip_ref_cacl], UD_ip_ref/1
  Constant3/1 -> Math Function/2
  Integrator/1 -> Math Function/1
  [Phi] -> MATLAB Function/4(theta)
  MATLAB Function/1(xD) -> UD/1, [UD]
  [Phi] -> MATLAB Function1/4(theta)
  Demux5/1 -> MATLAB Function1/1(xA)
  Demux5/2 -> MATLAB Function1/2(xB)
  Demux5/3 -> MATLAB Function1/3(xC)
  Imeas/1 -> Demux6/1
  MATLAB Function/2(xQ) -> Terminator1/1
  Demux6/1 -> MATLAB Function2/1(xA)
  Demux6/2 -> MATLAB Function2/2(xB)
  Demux6/3 -> MATLAB Function2/3(xC)
  [Phi] -> MATLAB Function2/4(theta)

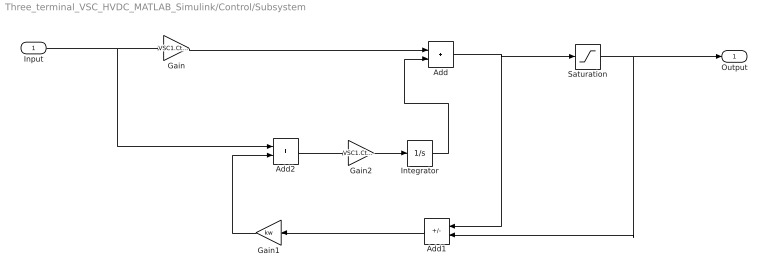
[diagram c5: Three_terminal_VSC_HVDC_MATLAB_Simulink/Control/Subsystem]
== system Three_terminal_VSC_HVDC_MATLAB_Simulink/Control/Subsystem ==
  Input : Inport
  Add : Sum
  Add1 : Sum  Inputs=-+
  Add2 : Sum
  Gain : Gain  Gain=VSC1.Ctrl.AC.Kp
  Gain1 : Gain  Gain=kw
  Gain2 : Gain  Gain=VSC1.Ctrl.AC.Ti
  Integrator : Integrator
  Saturation : Saturate  UpperLimit=VSC1.Ctrl.Iqmax  LowerLimit=VSC1.Ctrl.Iqmin
  Output : Outport
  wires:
  Gain/1 -> Add/1
  Input/1 -> Add2/1, Gain/1
  Add/1 -> Add1/1, Saturation/1
  Saturation/1 -> Add1/2, Output/1
  Add1/1 -> Gain1/1
  Gain1/1 -> Add2/2
  Add2/1 -> Gain2/1
  Gain2/1 -> Integrator/1
  Integrator/1 -> Add/2

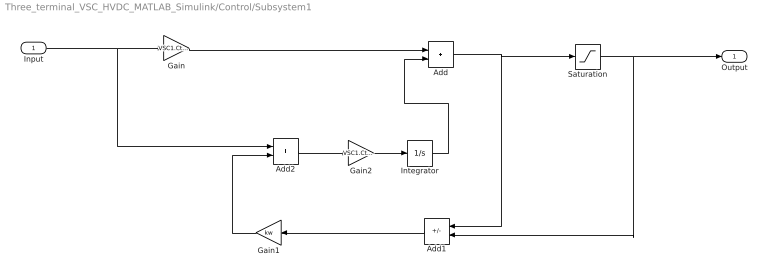
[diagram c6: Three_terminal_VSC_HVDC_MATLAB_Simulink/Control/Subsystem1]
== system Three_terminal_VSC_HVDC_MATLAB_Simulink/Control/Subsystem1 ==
  Input : Inport
  Add : Sum
  Add1 : Sum  Inputs=-+
  Add2 : Sum
  Gain : Gain  Gain=VSC1.Ctrl.DC.Kp
  Gain1 : Gain  Gain=kw
  Gain2 : Gain  Gain=VSC1.Ctrl.DC.Ti
  Integrator : Integrator
  Saturation : Saturate  UpperLimit=VSC1.Ctrl.Idmax  LowerLimit=VSC1.Ctrl.Idmin
  Output : Outport
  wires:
  Gain/1 -> Add/1
  Input/1 -> Add2/1, Gain/1
  Add/1 -> Add1/1, Saturation/1
  Saturation/1 -> Add1/2, Output/1
  Add1/1 -> Gain1/1
  Gain1/1 -> Add2/2
  Add2/1 -> Gain2/1
  Gain2/1 -> Integrator/1
  Integrator/1 -> Add/2

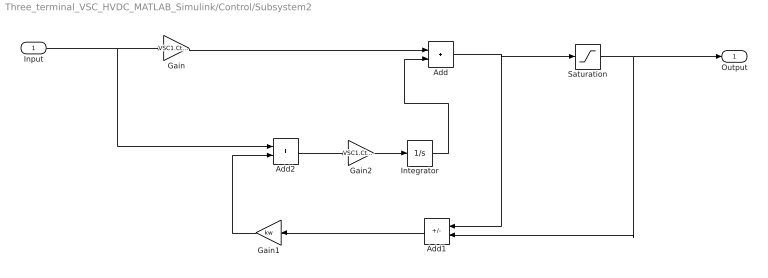
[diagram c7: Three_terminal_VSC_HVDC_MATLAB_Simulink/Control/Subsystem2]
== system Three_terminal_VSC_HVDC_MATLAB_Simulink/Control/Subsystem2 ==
  Input : Inport
  Add : Sum
  Add1 : Sum  Inputs=-+
  Add2 : Sum
  Gain : Gain  Gain=VSC1.Ctrl.Current.Kp
  Gain1 : Gain  Gain=kw
  Gain2 : Gain  Gain=VSC1.Ctrl.Current.Ti
  Integrator : Integrator
  Saturation : Saturate  UpperLimit=VSC1.Ctrl.Umax  LowerLimit=VSC1.Ctrl.Umin
  Output : Outport
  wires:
  Gain/1 -> Add/1
  Input/1 -> Add2/1, Gain/1
  Add/1 -> Add1/1, Saturation/1
  Saturation/1 -> Add1/2, Output/1
  Add1/1 -> Gain1/1
  Gain1/1 -> Add2/2
  Add2/1 -> Gain2/1
  Gain2/1 -> Integrator/1
  Integrator/1 -> Add/2

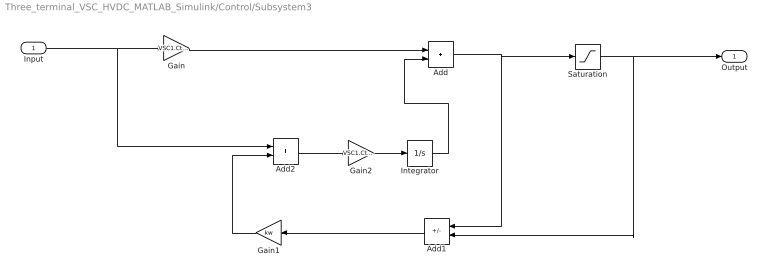
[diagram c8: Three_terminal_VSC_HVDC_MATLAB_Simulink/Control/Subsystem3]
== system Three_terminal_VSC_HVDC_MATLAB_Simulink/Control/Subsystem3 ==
  Input : Inport
  Add : Sum
  Add1 : Sum  Inputs=-+
  Add2 : Sum
  Gain : Gain  Gain=VSC1.Ctrl.Current.Kp
  Gain1 : Gain  Gain=kw
  Gain2 : Gain  Gain=VSC1.Ctrl.Current.Ti
  Integrator : Integrator
  Saturation : Saturate  UpperLimit=VSC1.Ctrl.Umax  LowerLimit=VSC1.Ctrl.Umin
  Output : Outport
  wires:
  Gain/1 -> Add/1
  Input/1 -> Add2/1, Gain/1
  Add/1 -> Add1/1, Saturation/1
  Saturation/1 -> Add1/2, Output/1
  Add1/1 -> Gain1/1
  Gain1/1 -> Add2/2
  Add2/1 -> Gain2/1
  Gain2/1 -> Integrator/1
  Integrator/1 -> Add/2

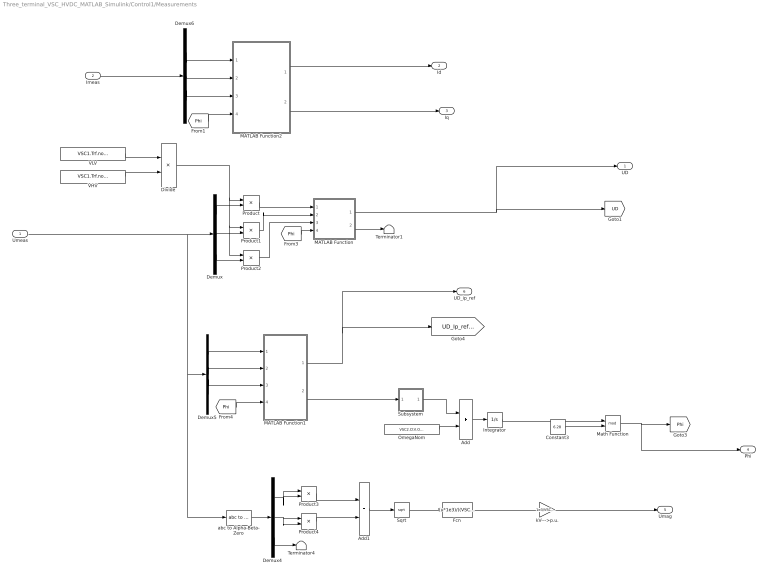
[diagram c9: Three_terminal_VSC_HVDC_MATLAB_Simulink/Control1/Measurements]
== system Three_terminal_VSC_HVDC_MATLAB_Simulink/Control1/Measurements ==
  Umeas : Inport
  Imeas : Inport  Port=2
  Add : Sum
  Add1 : Sum
  Constant3 : Constant  Value=6.28
  Demux{,4..6} (4 alike) : Demux  Outputs=3
  Divide : Product  Inputs=*/
  Fcn : Fcn  Expr=(u*1e3)/((VSC1.Trf.nominal.HV *sqrt(2))/(sqrt(3)*VSC1.Trf.nominal.HV ))/1000
  Integrator : Integrator
  MATLAB Function : MATLAB Function  TreatAsAtomicUnit=on
  MATLAB Function1 : MATLAB Function  TreatAsAtomicUnit=on
  MATLAB Function2 : MATLAB Function  TreatAsAtomicUnit=on
  Math Function : Math  Operator=mod
  OmegaNom : Constant  Value=VSC2.Ctrl.Omeganom
  Product{,1..4} (5 alike) : Product
  Sqrt : Sqrt
  Subsystem : Subsystem
  Terminator1 : Terminator
  Terminator4 : Terminator
  VHV : Constant  Value=VSC1.Trf.nominal.HV
  VLV : Constant  Value=VSC1.Trf.nominal.LV
  abc to Alpha-Beta-Zero : powerlib_meascontrol/Transformations/abc to Alpha-Beta-Zero
  kV--->p.u. : Gain  Gain=1e3/VSC1.Trf.nominal.HV
  UD : Outport
  Id : Outport  Port=2
  Iq : Outport  Port=3
  Phi : Outport  Port=4
  Umag : Outport  Port=5
  UD_ip_ref : Outport  Port=6
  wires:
  MATLAB Function1/2(xQ) -> Subsystem/1(Input)
  MATLAB Function2/2(xQ) -> Iq/1
  Demux/2 -> Product1/2
  Subsystem/1(Output) -> Add/1
  Math Function/1 -> Phi/1, [Phi]
  Product2/1 -> MATLAB Function/3(xC)
  Divide/1 -> Product/1, Product1/1, Product2/1
  Product/1 -> MATLAB Function/1(xA)
  VLV/1 -> Divide/1
  OmegaNom/1 -> Add/2
  Product1/1 -> MATLAB Function/2(xB)
  Add/1 -> Integrator/1
  VHV/1 -> Divide/2
  Demux/1 -> Product/2
  Demux/3 -> Product2/2
  MATLAB Function2/1(xD) -> Id/1
  abc to Alpha-Beta-Zero/1 -> Demux4/1
  Demux4/1 -> Product3/2, Product3/1
  Demux4/2 -> Product4/2, Product4/1
  Demux4/3 -> Terminator4/1
  Product3/1 -> Add1/1
  Product4/1 -> Add1/2
  Add1/1 -> Sqrt/1
  Sqrt/1 -> Fcn/1
  Fcn/1 -> kV--->p.u./1
  kV--->p.u./1 -> Umag/1
  Umeas/1 -> Demux/1, abc to Alpha-Beta-Zero/1, Demux5/1
  MATLAB Function1/1(xD) -> [UD_Ip_ref_cacl], UD_ip_ref/1
  Constant3/1 -> Math Function/2
  Integrator/1 -> Math Function/1
  [Phi] -> MATLAB Function/4(theta)
  MATLAB Function/1(xD) -> UD/1, [UD]
  [Phi] -> MATLAB Function1/4(theta)
  Demux5/1 -> MATLAB Function1/1(xA)
  Demux5/2 -> MATLAB Function1/2(xB)
  Demux5/3 -> MATLAB Function1/3(xC)
  Imeas/1 -> Demux6/1
  MATLAB Function/2(xQ) -> Terminator1/1
  Demux6/1 -> MATLAB Function2/1(xA)
  Demux6/2 -> MATLAB Function2/2(xB)
  Demux6/3 -> MATLAB Function2/3(xC)
  [Phi] -> MATLAB Function2/4(theta)

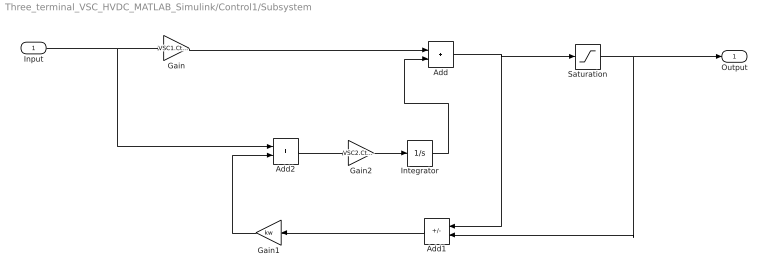
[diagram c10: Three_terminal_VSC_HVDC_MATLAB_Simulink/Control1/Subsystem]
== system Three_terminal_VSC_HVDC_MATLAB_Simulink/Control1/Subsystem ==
  Input : Inport
  Add : Sum
  Add1 : Sum  Inputs=-+
  Add2 : Sum
  Gain : Gain  Gain=VSC1.Ctrl.AC.Kp
  Gain1 : Gain  Gain=kw
  Gain2 : Gain  Gain=VSC2.Ctrl.AC.Ti
  Integrator : Integrator
  Saturation : Saturate  UpperLimit=VSC1.Ctrl.Iqmax  LowerLimit=VSC1.Ctrl.Iqmin
  Output : Outport
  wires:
  Gain/1 -> Add/1
  Input/1 -> Add2/1, Gain/1
  Add/1 -> Add1/1, Saturation/1
  Saturation/1 -> Add1/2, Output/1
  Add1/1 -> Gain1/1
  Gain1/1 -> Add2/2
  Add2/1 -> Gain2/1
  Gain2/1 -> Integrator/1
  Integrator/1 -> Add/2

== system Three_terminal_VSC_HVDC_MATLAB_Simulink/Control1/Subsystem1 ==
  Input : Inport
  Add : Sum
  Add1 : Sum  Inputs=-+
  Add2 : Sum
  Gain : Gain  Gain=VSC1.Ctrl.DC.Kp
  Gain1 : Gain  Gain=kw
  Gain2 : Gain  Gain=VSC2.Ctrl.DC.Ti
  Integrator : Integrator
  Saturation : Saturate  UpperLimit=VSC1.Ctrl.Idmax  LowerLimit=VSC1.Ctrl.Idmin
  Output : Outport
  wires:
  Gain/1 -> Add/1
  Input/1 -> Add2/1, Gain/1
  Add/1 -> Add1/1, Saturation/1
  Saturation/1 -> Add1/2, Output/1
  Add1/1 -> Gain1/1
  Gain1/1 -> Add2/2
  Add2/1 -> Gain2/1
  Gain2/1 -> Integrator/1
  Integrator/1 -> Add/2

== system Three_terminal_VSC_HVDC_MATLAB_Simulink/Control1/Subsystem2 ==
  Input : Inport
  Add : Sum
  Add1 : Sum  Inputs=-+
  Add2 : Sum
  Gain : Gain  Gain=VSC1.Ctrl.Current.Kp
  Gain1 : Gain  Gain=kw
  Gain2 : Gain  Gain=VSC1.Ctrl.Current.Ti
  Integrator : Integrator
  Saturation : Saturate  UpperLimit=VSC1.Ctrl.Umax  LowerLimit=VSC1.Ctrl.Umin
  Output : Outport
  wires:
  Gain/1 -> Add/1
  Input/1 -> Add2/1, Gain/1
  Add/1 -> Add1/1, Saturation/1
  Saturation/1 -> Add1/2, Output/1
  Add1/1 -> Gain1/1
  Gain1/1 -> Add2/2
  Add2/1 -> Gain2/1
  Gain2/1 -> Integrator/1
  Integrator/1 -> Add/2

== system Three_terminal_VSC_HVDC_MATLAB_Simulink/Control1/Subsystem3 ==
  Input : Inport
  Add : Sum
  Add1 : Sum  Inputs=-+
  Add2 : Sum
  Gain : Gain  Gain=VSC1.Ctrl.Current.Kp
  Gain1 : Gain  Gain=kw
  Gain2 : Gain  Gain=VSC1.Ctrl.Current.Ti
  Integrator : Integrator
  Saturation : Saturate  UpperLimit=VSC1.Ctrl.Umax  LowerLimit=VSC1.Ctrl.Umin
  Output : Outport
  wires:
  Gain/1 -> Add/1
  Input/1 -> Add2/1, Gain/1
  Add/1 -> Add1/1, Saturation/1
  Saturation/1 -> Add1/2, Output/1
  Add1/1 -> Gain1/1
  Gain1/1 -> Add2/2
  Add2/1 -> Gain2/1
  Gain2/1 -> Integrator/1
  Integrator/1 -> Add/2
